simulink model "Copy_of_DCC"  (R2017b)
settings: Solver=FixedStepDiscrete  StartTime=0.0  StopTime=10.0  FixedStep=0.01  RelTol=1e-3  EnableMultiTasking=on
undefined symbols (not defined in the file): ASWTYPE_FALSE, ASWTYPE_TRUE, CbDCC_BMTMsgCmd_flg, CbDCC_BMVMsgCmd_flg, CbDCC_BSPMsgCmd_flg, CcDCC_BSTSendTi_ms, CcDCC_BulkSOC_pct, CcDCC_CCSTout_ms, CcDCC_CellTempFilterAvg_numb, CcDCC_ChrgCrnt0HysVolt_mV, CcDCC_ChrgFinOverTi_ms, CcDCC_ChrgMaxPackVoltLimt_V, CcDCC_ChrgSt2StepChrgTime_ms, CcDCC_ChrgStCutoffTime_ms, CcDCC_ChrgStFullChrgCrnt_A, CcDCC_CMLTout_ms, CcDCC_CommToutOverTi_ms, CcDCC_CRMAATout_ms, CcDCC_CRMCHMTout_ms, CcDCC_CRMTout_ms, CcDCC_CROAATout_ms, CcDCC_CROTout_ms, CcDCC_CSDTout_ms, CcDCC_CSTTout_ms, CcDCC_DC12VUnonnectTi_ms, CcDCC_DCChrgDispSOCPrmt_pct, CcDCC_DCChrgMismatch_ms, CcDCC_DCChrgPermitCfg_ms, CcDCC_DCChrgPrmtFltLvl_numb, CcDCC_DCChrgPrmtStop_ms, CcDCC_DCChrgStepCurr_A, CcDCC_DCChrgStop_ms, CcDCC_DCCrntUnctrolTi_ms, CcDCC_DCFullChrgHysVolt_mV, CcDCC_DCFullStepChrgTi1_ms, CcDCC_DCFullStepChrgTi2_ms, CcDCC_DCMaxChrgCurr_A, CcDCC_DCStepChrgWaitTime_ms, CcDCC_DCStop2DefaultTi_ms, CcDCC_DefaultWaitTi_ms, CcDCC_DiffDCChrgCrnt_A, CcDCC_DiffDCChrgCrntTi_ms, CcDCC_HeatChrgCrnt0Time_ms, CcDCC_HeatChrgCrnt1Time_ms, CcDCC_IsoDisableDelay_ms, CcDCC_MaxPackVoltLimt_V, CcDCC_SafeCur_A, CcDCC_StartChrgHysVolt_mV, CcDCC_StartDCChrgCellTemp_C, CcDCC_StepChrgCutoffTi_ms, CcDCC_StepChrgFullChrgCrnt_A, CcDCC_ToutDelay_ms, CcDCC_VehSpdFld_kmh, DCC_CONST0_NUMB, DCC_CONST1000_NUMB, DCC_CONST170_NUMB, DCC_RUNTIME_MS, Enum_BTMHeatReq, Enum_CTCCtrCtlConnMode, Enum_CTCCtrCtlState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
libraries: AIWAYS_Powertrain_BMS_lib x82
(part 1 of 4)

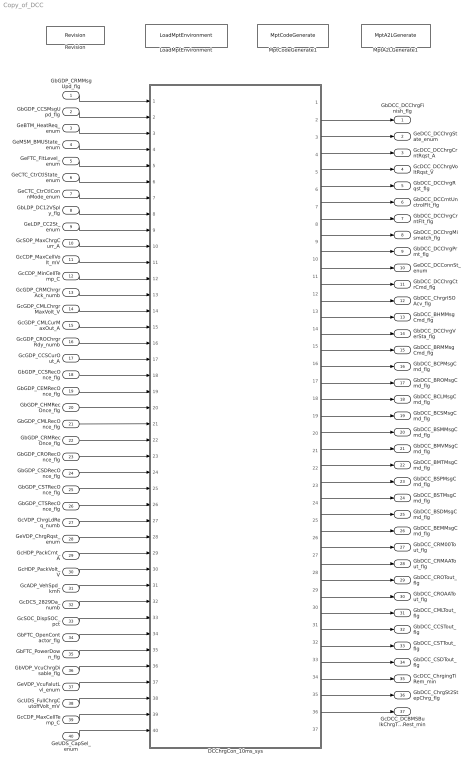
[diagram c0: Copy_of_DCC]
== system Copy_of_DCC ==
  GbGDP_CRMMsgUpd_flg : Inport
  GbGDP_CCSMsgUpd_flg : Inport  Port=2
  GeBTM_HeatReq_enum : Inport  Port=3
  GeMSM_BMUState_enum : Inport  Port=4
  GeFTC_FltLevel_enum : Inport  Port=5
  GeCTC_CtrCtlState_enum : Inport  Port=6
  GeCTC_CtrCtlConnMode_enum : Inport  Port=7
  GbLDP_DC12VSply_flg : Inport  Port=8
  GeLDP_CC2St_enum : Inport  Port=9
  GcSOP_MaxChrgCurr_A : Inport  Port=10
  GcCDP_MaxCellVolt_mV : Inport  Port=11
  GcCDP_MinCellTemp_C : Inport  Port=12
  GcGDP_CRMChrgrAck_numb : Inport  Port=13
  GcGDP_CMLChrgrMaxVolt_V : Inport  Port=14
  GcGDP_CMLCurMaxOut_A : Inport  Port=15
  GcGDP_CROChrgrRdy_numb : Inport  Port=16
  GcGDP_CCSCurOut_A : Inport  Port=17
  GbGDP_CCSRecOnce_flg : Inport  Port=18
  GbGDP_CEMRecOnce_flg : Inport  Port=19
  GbGDP_CHMRecOnce_flg : Inport  Port=20
  GbGDP_CMLRecOnce_flg : Inport  Port=21
  GbGDP_CRMRecOnce_flg : Inport  Port=22
  GbGDP_CRORecOnce_flg : Inport  Port=23
  GbGDP_CSDRecOnce_flg : Inport  Port=24
  GbGDP_CSTRecOnce_flg : Inport  Port=25
  GbGDP_CTSRecOnce_flg : Inport  Port=26
  GcVDP_ChrgLdReq_numb : Inport  Port=27
  GeVDP_ChrgRqst_enum : Inport  Port=28
  GcHDP_PackCrnt_A : Inport  Port=29
  GcHDP_PackVolt_V : Inport  Port=30
  GcADP_VehSpd_kmh : Inport  Port=31
  GcDCS_2829Da_numb : Inport  Port=32
  GcSOC_DispSOC_pct : Inport  Port=33
  GbFTC_OpenContactor_flg : Inport  Port=34
  GbFTC_PowerDown_flg : Inport  Port=35
  GbVDP_VcuChrgDisable_flg : Inport  Port=36
  GeVDP_VcuFalutLvl_enum : Inport  Port=37
  GcUDS_FullChrgCutoffVolt_mV : Inport  Port=38
  GcCDP_MaxCellTemp_C : Inport  Port=39
  GeUDS_CapSel_enum : Inport  Port=40
  DCChrgCon_10ms_sys : Subsystem
  LoadMptEnvironment : AIWAYS_Powertrain_BMS_lib/Config/LoadMptEnvironment  ProjectName=Comm  SuppierID=NewPlatformUAES
  MptA2LGenerate1 : AIWAYS_Powertrain_BMS_lib/Config/MptA2LGenerate  SystemSampleTime=-1
  MptCodeGenerate1 : AIWAYS_Powertrain_BMS_lib/Config/MptCodeGenerate  SystemSampleTime=-1
  Revision : AIWAYS_Powertrain_BMS_lib/Config/Revision  curVersion='M111C107'  newVersion='M112C107'
  GbDCC_DCChrgFinish_flg : Outport
  GeDCC_DCChrgState_enum : Outport  Port=2
  GcDCC_DCChrgCrntRqst_A : Outport  Port=3
  GcDCC_DCChrgVoltRqst_V : Outport  Port=4
  GbDCC_DCChrgRqst_flg : Outport  Port=5
  GbDCC_DCCrntUnctrolFlt_flg : Outport  Port=6
  GbDCC_DCChrgCrntFlt_flg : Outport  Port=7
  GbDCC_DCChrgMismatch_flg : Outport  Port=8
  GbDCC_DCChrgPrmt_flg : Outport  Port=9
  GeDCC_DCConnSt_enum : Outport  Port=10
  GbDCC_DCChrgCtrCmd_flg : Outport  Port=11
  GbDCC_ChrgrISOAcv_flg : Outport  Port=12
  GbDCC_BHMMsgCmd_flg : Outport  Port=13
  GbDCC_DCChrgVerSta_flg : Outport  Port=14
  GbDCC_BRMMsgCmd_flg : Outport  Port=15
  GbDCC_BCPMsgCmd_flg : Outport  Port=16
  GbDCC_BROMsgCmd_flg : Outport  Port=17
  GbDCC_BCLMsgCmd_flg : Outport  Port=18
  GbDCC_BCSMsgCmd_flg : Outport  Port=19
  GbDCC_BSMMsgCmd_flg : Outport  Port=20
  GbDCC_BMVMsgCmd_flg : Outport  Port=21
  GbDCC_BMTMsgCmd_flg : Outport  Port=22
  GbDCC_BSPMsgCmd_flg : Outport  Port=23
  GbDCC_BSTMsgCmd_flg : Outport  Port=24
  GbDCC_BSDMsgCmd_flg : Outport  Port=25
  GbDCC_BEMMsgCmd_flg : Outport  Port=26
  GbDCC_CRM00Tout_flg : Outport  Port=27
  GbDCC_CRMAATout_flg : Outport  Port=28
  GbDCC_CROTout_flg : Outport  Port=29
  GbDCC_CROAATout_flg : Outport  Port=30
  GbDCC_CMLTout_flg : Outport  Port=31
  GbDCC_CCSTout_flg : Outport  Port=32
  GbDCC_CSTTout_flg : Outport  Port=33
  GbDCC_CSDTout_flg : Outport  Port=34
  GcDCC_ChrgingTiRem_min : Outport  Port=35
  GbDCC_ChrgSt2StepChrg_flg : Outport  Port=36
  GcDCC_DCBMSBulkChrgTimeRest_min : Outport  Port=37
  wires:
  DCChrgCon_10ms_sys/1(GbDCC_DCChrgFinish_flg) -> GbDCC_DCChrgFinish_flg/1
  DCChrgCon_10ms_sys/3(GcDCC_DCChrgCrntRqst_A) -> GcDCC_DCChrgCrntRqst_A/1
  DCChrgCon_10ms_sys/2(GeDCC_DCChrgState_enum) -> GeDCC_DCChrgState_enum/1
  DCChrgCon_10ms_sys/7(GbDCC_DCChrgCrntFlt_flg) -> GbDCC_DCChrgCrntFlt_flg/1
  DCChrgCon_10ms_sys/4(GcDCC_DCChrgVoltRqst_V) -> GcDCC_DCChrgVoltRqst_V/1
  DCChrgCon_10ms_sys/10(GeDCC_DCConnSt_enum) -> GeDCC_DCConnSt_enum/1
  DCChrgCon_10ms_sys/12(GbDCC_ChrgrISOAcv_flg) -> GbDCC_ChrgrISOAcv_flg/1
  DCChrgCon_10ms_sys/15(GbDCC_BRMMsgCmd_flg) -> GbDCC_BRMMsgCmd_flg/1
  DCChrgCon_10ms_sys/16(GbDCC_BCPMsgCmd_flg) -> GbDCC_BCPMsgCmd_flg/1
  GeLDP_CC2St_enum/1 -> DCChrgCon_10ms_sys/9(GeLDP_CC2St_enum)
  DCChrgCon_10ms_sys/11(GbDCC_DCChrgCtrCmd_flg) -> GbDCC_DCChrgCtrCmd_flg/1
  GcSOP_MaxChrgCurr_A/1 -> DCChrgCon_10ms_sys/10(GcSOP_MaxChrgCurr_A)
  GcCDP_MinCellTemp_C/1 -> DCChrgCon_10ms_sys/12(GcCDP_MinCellTemp_C)
  GcGDP_CMLChrgrMaxVolt_V/1 -> DCChrgCon_10ms_sys/14(GcGDP_CMLChrgrMaxVolt_V)
  GeBTM_HeatReq_enum/1 -> DCChrgCon_10ms_sys/3(GeBTM_HeatReq_enum)
  DCChrgCon_10ms_sys/5(GbDCC_DCChrgRqst_flg) -> GbDCC_DCChrgRqst_flg/1
  DCChrgCon_10ms_sys/25(GbDCC_BSDMsgCmd_flg) -> GbDCC_BSDMsgCmd_flg/1
  GeUDS_CapSel_enum/1 -> DCChrgCon_10ms_sys/40(GeUDS_CapSel_enum)
  GcGDP_CROChrgrRdy_numb/1 -> DCChrgCon_10ms_sys/16(GcGDP_CROChrgrRdy_numb)
  GbGDP_CRMMsgUpd_flg/1 -> DCChrgCon_10ms_sys/1(GbGDP_CRMMsgUpd_flg)
  DCChrgCon_10ms_sys/22(GbDCC_BMTMsgCmd_flg) -> GbDCC_BMTMsgCmd_flg/1
  GcGDP_CCSCurOut_A/1 -> DCChrgCon_10ms_sys/17(GcGDP_CCSCurOut_A)
  DCChrgCon_10ms_sys/30(GbDCC_CROAATout_flg) -> GbDCC_CROAATout_flg/1
  GbGDP_CMLRecOnce_flg/1 -> DCChrgCon_10ms_sys/21(GbGDP_CMLRecOnce_flg)
  DCChrgCon_10ms_sys/14(GbDCC_DCChrgVerSta_flg) -> GbDCC_DCChrgVerSta_flg/1
  GbGDP_CRORecOnce_flg/1 -> DCChrgCon_10ms_sys/23(GbGDP_CRORecOnce_flg)
  DCChrgCon_10ms_sys/32(GbDCC_CCSTout_flg) -> GbDCC_CCSTout_flg/1
  DCChrgCon_10ms_sys/17(GbDCC_BROMsgCmd_flg) -> GbDCC_BROMsgCmd_flg/1
  GeFTC_FltLevel_enum/1 -> DCChrgCon_10ms_sys/5(GeFTC_FltLevel_enum)
  DCChrgCon_10ms_sys/27(GbDCC_CRM00Tout_flg) -> GbDCC_CRM00Tout_flg/1
  DCChrgCon_10ms_sys/13(GbDCC_BHMMsgCmd_flg) -> GbDCC_BHMMsgCmd_flg/1
  DCChrgCon_10ms_sys/28(GbDCC_CRMAATout_flg) -> GbDCC_CRMAATout_flg/1
  GcCDP_MaxCellVolt_mV/1 -> DCChrgCon_10ms_sys/11(GcCDP_MaxCellVolt_mV)
  GbLDP_DC12VSply_flg/1 -> DCChrgCon_10ms_sys/8(GbLDP_DC12VSply_flg)
  DCChrgCon_10ms_sys/20(GbDCC_BSMMsgCmd_flg) -> GbDCC_BSMMsgCmd_flg/1
  DCChrgCon_10ms_sys/24(GbDCC_BSTMsgCmd_flg) -> GbDCC_BSTMsgCmd_flg/1
  GeVDP_VcuFalutLvl_enum/1 -> DCChrgCon_10ms_sys/37(GeVDP_VcuFalutLvl_enum)
  GcVDP_ChrgLdReq_numb/1 -> DCChrgCon_10ms_sys/27(GcVDP_ChrgLdReq_numb)
  GcHDP_PackCrnt_A/1 -> DCChrgCon_10ms_sys/29(GcHDP_PackCrnt_A)
  GcCDP_MaxCellTemp_C/1 -> DCChrgCon_10ms_sys/39(GcCDP_MaxCellTemp_C)
  GbGDP_CCSRecOnce_flg/1 -> DCChrgCon_10ms_sys/18(GbGDP_CCSRecOnce_flg)
  GcDCS_2829Da_numb/1 -> DCChrgCon_10ms_sys/32(GcDCS_2829Da_numb)
  GcADP_VehSpd_kmh/1 -> DCChrgCon_10ms_sys/31(GcADP_VehSpd_kmh)
  DCChrgCon_10ms_sys/37(GcDCC_DCBMSBulkChrgTimeRest_min) -> GcDCC_DCBMSBulkChrgTimeRest_min/1
  DCChrgCon_10ms_sys/23(GbDCC_BSPMsgCmd_flg) -> GbDCC_BSPMsgCmd_flg/1
  GbGDP_CSTRecOnce_flg/1 -> DCChrgCon_10ms_sys/25(GbGDP_CSTRecOnce_flg)
  DCChrgCon_10ms_sys/21(GbDCC_BMVMsgCmd_flg) -> GbDCC_BMVMsgCmd_flg/1
  GcSOC_DispSOC_pct/1 -> DCChrgCon_10ms_sys/33(GcSOC_DispSOC_pct)
  DCChrgCon_10ms_sys/9(GbDCC_DCChrgPrmt_flg) -> GbDCC_DCChrgPrmt_flg/1
  GcUDS_FullChrgCutoffVolt_mV/1 -> DCChrgCon_10ms_sys/38(GcUDS_FullChrgCutoffVolt_mV)
  DCChrgCon_10ms_sys/35(GcDCC_ChrgingTiRem_min) -> GcDCC_ChrgingTiRem_min/1
  DCChrgCon_10ms_sys/36(GbDCC_ChrgSt2StepChrg_flg) -> GbDCC_ChrgSt2StepChrg_flg/1
  GeVDP_ChrgRqst_enum/1 -> DCChrgCon_10ms_sys/28(GeVDP_ChrgRqst_enum)
  GbGDP_CRMRecOnce_flg/1 -> DCChrgCon_10ms_sys/22(GbGDP_CRMRecOnce_flg)
  GcHDP_PackVolt_V/1 -> DCChrgCon_10ms_sys/30(GcHDP_PackVolt_V)
  DCChrgCon_10ms_sys/31(GbDCC_CMLTout_flg) -> GbDCC_CMLTout_flg/1
  GbGDP_CEMRecOnce_flg/1 -> DCChrgCon_10ms_sys/19(GbGDP_CEMRecOnce_flg)
  GeCTC_CtrCtlState_enum/1 -> DCChrgCon_10ms_sys/6(GeCTC_CtrCtlState_enum)
  GbGDP_CCSMsgUpd_flg/1 -> DCChrgCon_10ms_sys/2(GbGDP_CCSMsgUpd_flg)
  GbFTC_PowerDown_flg/1 -> DCChrgCon_10ms_sys/35(GbFTC_PowerDown_flg)
  DCChrgCon_10ms_sys/26(GbDCC_BEMMsgCmd_flg) -> GbDCC_BEMMsgCmd_flg/1
  GbGDP_CSDRecOnce_flg/1 -> DCChrgCon_10ms_sys/24(GbGDP_CSDRecOnce_flg)
  GbGDP_CTSRecOnce_flg/1 -> DCChrgCon_10ms_sys/26(GbGDP_CTSRecOnce_flg)
  GcGDP_CMLCurMaxOut_A/1 -> DCChrgCon_10ms_sys/15(GcGDP_CMLCurMaxOut_A)
  GbGDP_CHMRecOnce_flg/1 -> DCChrgCon_10ms_sys/20(GbGDP_CHMRecOnce_flg)
  DCChrgCon_10ms_sys/6(GbDCC_DCCrntUnctrolFlt_flg) -> GbDCC_DCCrntUnctrolFlt_flg/1
  DCChrgCon_10ms_sys/29(GbDCC_CROTout_flg) -> GbDCC_CROTout_flg/1
  DCChrgCon_10ms_sys/34(GbDCC_CSDTout_flg) -> GbDCC_CSDTout_flg/1
  GbVDP_VcuChrgDisable_flg/1 -> DCChrgCon_10ms_sys/36(GbVDP_VcuChrgDisable_flg)
  DCChrgCon_10ms_sys/19(GbDCC_BCSMsgCmd_flg) -> GbDCC_BCSMsgCmd_flg/1
  GeCTC_CtrCtlConnMode_enum/1 -> DCChrgCon_10ms_sys/7(GeCTC_CtrCtlConnMode_enum)
  DCChrgCon_10ms_sys/18(GbDCC_BCLMsgCmd_flg) -> GbDCC_BCLMsgCmd_flg/1
  GeMSM_BMUState_enum/1 -> DCChrgCon_10ms_sys/4(GeMSM_BMUState_enum)
  GbFTC_OpenContactor_flg/1 -> DCChrgCon_10ms_sys/34(GbFTC_OpenContactor_flg)
  GcGDP_CRMChrgrAck_numb/1 -> DCChrgCon_10ms_sys/13(GcGDP_CRMChrgrAck_numb)
  DCChrgCon_10ms_sys/33(GbDCC_CSTTout_flg) -> GbDCC_CSTTout_flg/1
  DCChrgCon_10ms_sys/8(GbDCC_DCChrgMismatch_flg) -> GbDCC_DCChrgMismatch_flg/1

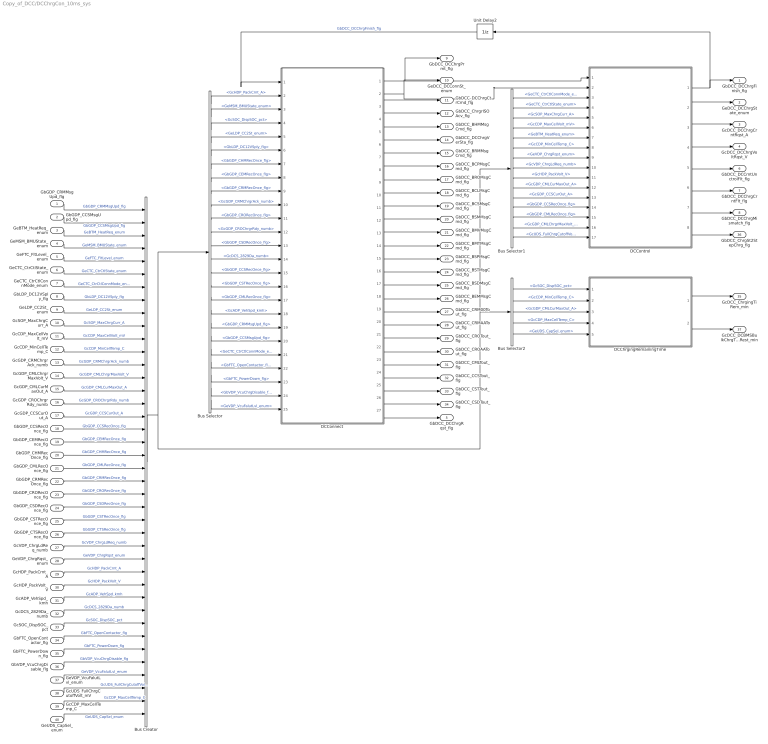
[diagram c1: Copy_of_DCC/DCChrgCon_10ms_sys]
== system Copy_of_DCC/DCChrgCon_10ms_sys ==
  GbGDP_CRMMsgUpd_flg : Inport
  GbGDP_CCSMsgUpd_flg : Inport  Port=2
  GeBTM_HeatReq_enum : Inport  Port=3
  GeMSM_BMUState_enum : Inport  Port=4
  GeFTC_FltLevel_enum : Inport  Port=5
  GeCTC_CtrCtlState_enum : Inport  Port=6
  GeCTC_CtrCtlConnMode_enum : Inport  Port=7
  GbLDP_DC12VSply_flg : Inport  Port=8
  GeLDP_CC2St_enum : Inport  Port=9
  GcSOP_MaxChrgCurr_A : Inport  Port=10
  GcCDP_MaxCellVolt_mV : Inport  Port=11
  GcCDP_MinCellTemp_C : Inport  Port=12
  GcGDP_CRMChrgrAck_numb : Inport  Port=13
  GcGDP_CMLChrgrMaxVolt_V : Inport  Port=14
  GcGDP_CMLCurMaxOut_A : Inport  Port=15
  GcGDP_CROChrgrRdy_numb : Inport  Port=16
  GcGDP_CCSCurOut_A : Inport  Port=17
  GbGDP_CCSRecOnce_flg : Inport  Port=18
  GbGDP_CEMRecOnce_flg : Inport  Port=19
  GbGDP_CHMRecOnce_flg : Inport  Port=20
  GbGDP_CMLRecOnce_flg : Inport  Port=21
  GbGDP_CRMRecOnce_flg : Inport  Port=22
  GbGDP_CRORecOnce_flg : Inport  Port=23
  GbGDP_CSDRecOnce_flg : Inport  Port=24
  GbGDP_CSTRecOnce_flg : Inport  Port=25
  GbGDP_CTSRecOnce_flg : Inport  Port=26
  GcVDP_ChrgLdReq_numb : Inport  Port=27
  GeVDP_ChrgRqst_enum : Inport  Port=28
  GcHDP_PackCrnt_A : Inport  Port=29
  GcHDP_PackVolt_V : Inport  Port=30
  GcADP_VehSpd_kmh : Inport  Port=31
  GcDCS_2829Da_numb : Inport  Port=32
  GcSOC_DispSOC_pct : Inport  Port=33
  GbFTC_OpenContactor_flg : Inport  Port=34
  GbFTC_PowerDown_flg : Inport  Port=35
  GbVDP_VcuChrgDisable_flg : Inport  Port=36
  GeVDP_VcuFalutLvl_enum : Inport  Port=37
  GcUDS_FullChrgCutoffVolt_mV : Inport  Port=38
  GcCDP_MaxCellTemp_C : Inport  Port=39
  GeUDS_CapSel_enum : Inport  Port=40
  Bus Creator : BusCreator  Inputs=40
  Bus Selector : BusSelector  OutputSignals=GcHDP_PackCrnt_A,GeMSM_BMUState_enum,GcSOC_DispSOC_pct,GeLDP_CC2St_enum,GbLDP_DC12VSply_flg,GbGDP_CHMRecOnce_flg,GbGDP_CEMRecOnce_flg,GbGDP_CRMRecOnce_flg,GcGDP_CRMChrgrAck_numb,GbGDP_CRORecOnce_flg,GcGDP_CROChrgrRdy_numb,GbGDP_CSDRecOnce_flg,GcDCS_2829Da_numb,GbGDP_CCSRecOnce_flg,GbGDP_CSTRecOnce_flg,GbGDP_CMLRecOnce_flg,GcADP_VehSpd_kmh,GbGDP_CRMMsgUpd_flg,GbGDP_CCSMsgUpd_flg,GeCTC_CtrCtlConnMod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
  Bus Selector1 : BusSelector  OutputSignals=GeCTC_CtrCtlConnMode_enum,GeCTC_CtrCtlState_enum,GcSOP_MaxChrgCurr_A,GcCDP_MaxCellVolt_mV,GeBTM_HeatReq_enum,GcCDP_MinCellTemp_C,GeVDP_ChrgRqst_enum,GcVDP_ChrgLdReq_numb,GcHDP_PackVolt_V,GcGDP_CMLCurMaxOut_A,GcGDP_CCSCurOut_A,GbGDP_CCSRecOnce_flg,GbGDP_CMLRecOnce_flg,GcGDP_CMLChrgrMaxVolt_V,GcUDS_FullChrgCutoffVolt_mV
  Bus Selector2 : BusSelector  OutputSignals=GcSOC_DispSOC_pct,GcCDP_MinCellTemp_C,GcGDP_CMLCurMaxOut_A,GcCDP_MaxCellTemp_C,GeUDS_CapSel_enum
  DCChrgingRemainingTime : Subsystem
  DCConnect : Subsystem
  DCControl : Subsystem
  Unit Delay2 : UnitDelay  SampleTime=-1  StateName=StateName
  GbDCC_DCChrgFinish_flg : Outport
  GeDCC_DCChrgState_enum : Outport  Port=2
  GcDCC_DCChrgCrntRqst_A : Outport  Port=3
  GcDCC_DCChrgVoltRqst_V : Outport  Port=4
  GbDCC_DCChrgRqst_flg : Outport  Port=5
  GbDCC_DCCrntUnctrolFlt_flg : Outport  Port=6
  GbDCC_DCChrgCrntFlt_flg : Outport  Port=7
  GbDCC_DCChrgMismatch_flg : Outport  Port=8
  GbDCC_DCChrgPrmt_flg : Outport  Port=9
  GeDCC_DCConnSt_enum : Outport  Port=10
  GbDCC_DCChrgCtrCmd_flg : Outport  Port=11
  GbDCC_ChrgrISOAcv_flg : Outport  Port=12
  GbDCC_BHMMsgCmd_flg : Outport  Port=13
  GbDCC_DCChrgVerSta_flg : Outport  Port=14
  GbDCC_BRMMsgCmd_flg : Outport  Port=15
  GbDCC_BCPMsgCmd_flg : Outport  Port=16
  GbDCC_BROMsgCmd_flg : Outport  Port=17
  GbDCC_BCLMsgCmd_flg : Outport  Port=18
  GbDCC_BCSMsgCmd_flg : Outport  Port=19
  GbDCC_BSMMsgCmd_flg : Outport  Port=20
  GbDCC_BMVMsgCmd_flg : Outport  Port=21
  GbDCC_BMTMsgCmd_flg : Outport  Port=22
  GbDCC_BSPMsgCmd_flg : Outport  Port=23
  GbDCC_BSTMsgCmd_flg : Outport  Port=24
  GbDCC_BSDMsgCmd_flg : Outport  Port=25
  GbDCC_BEMMsgCmd_flg : Outport  Port=26
  GbDCC_CRM00Tout_flg : Outport  Port=27
  GbDCC_CRMAATout_flg : Outport  Port=28
  GbDCC_CROTout_flg : Outport  Port=29
  GbDCC_CROAATout_flg : Outport  Port=30
  GbDCC_CMLTout_flg : Outport  Port=31
  GbDCC_CCSTout_flg : Outport  Port=32
  GbDCC_CSTTout_flg : Outport  Port=33
  GbDCC_CSDTout_flg : Outport  Port=34
  GcDCC_ChrgingTiRem_min : Outport  Port=35
  GbDCC_ChrgSt2StepChrg_flg : Outport  Port=36
  GcDCC_DCBMSBulkChrgTimeRest_min : Outport  Port=37
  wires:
  GbGDP_CRMMsgUpd_flg/1 -> Bus Creator/1  "GbGDP_CRMMsgUpd_flg"
  GbGDP_CCSMsgUpd_flg/1 -> Bus Creator/2  "GbGDP_CCSMsgUpd_flg"
  GeBTM_HeatReq_enum/1 -> Bus Creator/3  "GeBTM_HeatReq_enum"
  GeMSM_BMUState_enum/1 -> Bus Creator/4  "GeMSM_BMUState_enum"
  GeFTC_FltLevel_enum/1 -> Bus Creator/5  "GeFTC_FltLevel_enum"
  GeCTC_CtrCtlState_enum/1 -> Bus Creator/6  "GeCTC_CtrCtlState_enum"
  GeCTC_CtrCtlConnMode_enum/1 -> Bus Creator/7  "GeCTC_CtrCtlConnMode_enum"
  GbLDP_DC12VSply_flg/1 -> Bus Creator/8  "GbLDP_DC12VSply_flg"
  GeLDP_CC2St_enum/1 -> Bus Creator/9  "GeLDP_CC2St_enum"
  GcSOP_MaxChrgCurr_A/1 -> Bus Creator/10  "GcSOP_MaxChrgCurr_A"
  GcCDP_MaxCellVolt_mV/1 -> Bus Creator/11  "GcCDP_MaxCellVolt_mV"
  GcCDP_MinCellTemp_C/1 -> Bus Creator/12  "GcCDP_MinCellTemp_C"
  GcGDP_CRMChrgrAck_numb/1 -> Bus Creator/13  "GcGDP_CRMChrgrAck_numb"
  GcGDP_CMLChrgrMaxVolt_V/1 -> Bus Creator/14  "GcGDP_CMLChrgrMaxVolt_V"
  GcGDP_CMLCurMaxOut_A/1 -> Bus Creator/15  "GcGDP_CMLCurMaxOut_A"
  GcGDP_CROChrgrRdy_numb/1 -> Bus Creator/16  "GcGDP_CROChrgrRdy_numb"
  GcGDP_CCSCurOut_A/1 -> Bus Creator/17  "GcGDP_CCSCurOut_A"
  GbGDP_CCSRecOnce_flg/1 -> Bus Creator/18  "GbGDP_CCSRecOnce_flg"
  GbGDP_CEMRecOnce_flg/1 -> Bus Creator/19  "GbGDP_CEMRecOnce_flg"
  GbGDP_CHMRecOnce_flg/1 -> Bus Creator/20  "GbGDP_CHMRecOnce_flg"
  GbGDP_CMLRecOnce_flg/1 -> Bus Creator/21  "GbGDP_CMLRecOnce_flg"
  GbGDP_CRMRecOnce_flg/1 -> Bus Creator/22  "GbGDP_CRMRecOnce_flg"
  GbGDP_CRORecOnce_flg/1 -> Bus Creator/23  "GbGDP_CRORecOnce_flg"
  GbGDP_CSDRecOnce_flg/1 -> Bus Creator/24  "GbGDP_CSDRecOnce_flg"
  GbGDP_CSTRecOnce_flg/1 -> Bus Creator/25  "GbGDP_CSTRecOnce_flg"
  GbGDP_CTSRecOnce_flg/1 -> Bus Creator/26  "GbGDP_CTSRecOnce_flg"
  GcVDP_ChrgLdReq_numb/1 -> Bus Creator/27  "GcVDP_ChrgLdReq_numb"
  GeVDP_ChrgRqst_enum/1 -> Bus Creator/28  "GeVDP_ChrgRqst_enum"
  GcHDP_PackCrnt_A/1 -> Bus Creator/29  "GcHDP_PackCrnt_A"
  GcHDP_PackVolt_V/1 -> Bus Creator/30  "GcHDP_PackVolt_V"
  GcADP_VehSpd_kmh/1 -> Bus Creator/31  "GcADP_VehSpd_kmh"
  GcDCS_2829Da_numb/1 -> Bus Creator/32  "GcDCS_2829Da_numb"
  Bus Creator/1 -> Bus Selector/1, Bus Selector1/1, Bus Selector2/1
  GcSOC_DispSOC_pct/1 -> Bus Creator/33  "GcSOC_DispSOC_pct"
  DCControl/2(GeDCC_DCChrgState_enum) -> GeDCC_DCChrgState_enum/1
  DCControl/3(GcDCC_DCChrgCrntRqst_A) -> GcDCC_DCChrgCrntRqst_A/1
  DCControl/4(GcDCC_DCChrgVoltRqst_V) -> GcDCC_DCChrgVoltRqst_V/1
  DCControl/5(GbDCC_DCCrntUnctrolFlt_flg) -> GbDCC_DCCrntUnctrolFlt_flg/1
  DCControl/6(GbDCC_DCChrgCrntFlt_flg) -> GbDCC_DCChrgCrntFlt_flg/1
  DCControl/7(GbDCC_DCChrgMismatch_flg) -> GbDCC_DCChrgMismatch_flg/1
  DCControl/1(GbDCC_DCChrgFinish_flg) -> Unit Delay2/1, GbDCC_DCChrgFinish_flg/1
  Bus Selector/1 -> DCConnect/2(GcHDP_PackCrnt_A)  "<GcHDP_PackCrnt_A>"
  Bus Selector/2 -> DCConnect/3(GeMSM_BMUState_enum)  "<GeMSM_BMUState_enum>"
  Bus Selector/3 -> DCConnect/4(GcSOC_DispSOC_pct)  "<GcSOC_DispSOC_pct>"
  Bus Selector/6 -> DCConnect/7(GbGDP_CHMRecOnce_flg)  "<GbGDP_CHMRecOnce_flg>"
  Bus Selector/7 -> DCConnect/8(GbGDP_CEMRecOnce_flg)  "<GbGDP_CEMRecOnce_flg>"
  Bus Selector/8 -> DCConnect/9(GbGDP_CRMRecOnce_flg)  "<GbGDP_CRMRecOnce_flg>"
  Bus Selector/9 -> DCConnect/10(GcGDP_CRMChrgrAck_numb)  "<GcGDP_CRMChrgrAck_numb>"
  Bus Selector/10 -> DCConnect/11(GbGDP_CRORecOnce_flg)  "<GbGDP_CRORecOnce_flg>"
  Bus Selector/11 -> DCConnect/12(GcGDP_CROChrgrRdy_numb)  "<GcGDP_CROChrgrRdy_numb>"
  Bus Selector/12 -> DCConnect/13(GbGDP_CSDRecOnce_flg)  "<GbGDP_CSDRecOnce_flg>"
  Bus Selector/13 -> DCConnect/14(GcDCS_2829Da_numb)  "<GcDCS_2829Da_numb>"
  Bus Selector/14 -> DCConnect/15(GbGDP_CCSRecOnce_flg)  "<GbGDP_CCSRecOnce_flg>"
  Bus Selector/15 -> DCConnect/16(GbGDP_CSTRecOnce_flg)  "<GbGDP_CSTRecOnce_flg>"
  Bus Selector/16 -> DCConnect/17(GbGDP_CMLRecOnce_flg)  "<GbGDP_CMLRecOnce_flg>"
  Bus Selector/17 -> DCConnect/18(GcADP_VehSpd_kmh)  "<GcADP_VehSpd_kmh>"
  Bus Selector/18 -> DCConnect/19(GbGDP_CRMMsgUpd_flg)  "<GbGDP_CRMMsgUpd_flg>"
  Bus Selector/19 -> DCConnect/20(GbGDP_CCSMsgUpd_flg)  "<GbGDP_CCSMsgUpd_flg>"
  DCConnect/1(GbDCC_DCChrgPrmt_flg) -> GbDCC_DCChrgPrmt_flg/1, DCControl/1(GbDCC_DCChrgPrmt_flg)
  DCConnect/2(GeDCC_DCConnSt_enum) -> GeDCC_DCConnSt_enum/1, DCControl/2(GeDCC_DCConnSt_enum)
  Bus Selector1/1 -> DCControl/3(GeCTC_CtrCtlConnMode_enum)  "<GeCTC_CtrCtlConnMode_enum>"
  Bus Selector1/2 -> DCControl/4(GeCTC_CtrCtlState_enum)  "<GeCTC_CtrCtlState_enum>"
  Bus Selector1/3 -> DCControl/5(GcSOP_MaxChrgCurr_A)  "<GcSOP_MaxChrgCurr_A>"
  Bus Selector1/4 -> DCControl/6(GcCDP_MaxCellVolt_mV)  "<GcCDP_MaxCellVolt_mV>"
  Bus Selector1/5 -> DCControl/7(GeBTM_HeatReq_enum)  "<GeBTM_HeatReq_enum>"
  Bus Selector1/6 -> DCControl/8(GcCDP_MinCellTemp_C)  "<GcCDP_MinCellTemp_C>"
  Bus Selector1/7 -> DCControl/9(GeVDP_ChrgRqst_enum)  "<GeVDP_ChrgRqst_enum>"
  Bus Selector1/8 -> DCControl/10(GcVDP_ChrgLdReq_numb)  "<GcVDP_ChrgLdReq_numb>"
  Bus Selector1/9 -> DCControl/11(GcHDP_PackVolt_V)  "<GcHDP_PackVolt_V>"
  Bus Selector1/10 -> DCControl/12(GcGDP_CMLCurMaxOut_A)  "<GcGDP_CMLCurMaxOut_A>"
  Bus Selector1/11 -> DCControl/13(GcGDP_CCSCurOut_A)  "<GcGDP_CCSCurOut_A>"
  Bus Selector1/12 -> DCControl/14(GbGDP_CCSRecOnce_flg)  "<GbGDP_CCSRecOnce_flg>"
  Bus Selector1/13 -> DCControl/15(GbGDP_CMLRecOnce_flg)  "<GbGDP_CMLRecOnce_flg>"
  Bus Selector1/14 -> DCControl/16(GcGDP_CMLChrgrMaxVolt_V)  "<GcGDP_CMLChrgrMaxVolt_V>"
  DCConnect/3(GbDCC_DCChrgCtrCmd_flg) -> GbDCC_DCChrgCtrCmd_flg/1
  DCConnect/4(GbDCC_ChrgrISOAcv_flg) -> GbDCC_ChrgrISOAcv_flg/1
  DCConnect/5(GbDCC_BHMMsgCmd_flg) -> GbDCC_BHMMsgCmd_flg/1
  DCConnect/6(GbDCC_DCChrgVerSta_flg) -> GbDCC_DCChrgVerSta_flg/1
  DCConnect/7(GbDCC_BRMMsgCmd_flg) -> GbDCC_BRMMsgCmd_flg/1
  DCConnect/8(GbDCC_BCPMsgCmd_flg) -> GbDCC_BCPMsgCmd_flg/1
  DCConnect/9(GbDCC_BROMsgCmd_flg) -> GbDCC_BROMsgCmd_flg/1
  DCConnect/10(GbDCC_BCLMsgCmd_flg) -> GbDCC_BCLMsgCmd_flg/1
  DCConnect/11(GbDCC_BCSMsgCmd_flg) -> GbDCC_BCSMsgCmd_flg/1
  DCConnect/12(GbDCC_BSMMsgCmd_flg) -> GbDCC_BSMMsgCmd_flg/1
  DCConnect/13(GbDCC_BMVMsgCmd_flg) -> GbDCC_BMVMsgCmd_flg/1
  DCConnect/14(GbDCC_BMTMsgCmd_flg) -> GbDCC_BMTMsgCmd_flg/1
  DCConnect/15(GbDCC_BSPMsgCmd_flg) -> GbDCC_BSPMsgCmd_flg/1
  DCConnect/16(GbDCC_BSTMsgCmd_flg) -> GbDCC_BSTMsgCmd_flg/1
  DCConnect/17(GbDCC_BSDMsgCmd_flg) -> GbDCC_BSDMsgCmd_flg/1
  DCConnect/18(GbDCC_BEMMsgCmd_flg) -> GbDCC_BEMMsgCmd_flg/1
  DCConnect/19(GbDCC_CRM00Tout_flg) -> GbDCC_CRM00Tout_flg/1
  DCConnect/20(GbDCC_CRMAATout_flg) -> GbDCC_CRMAATout_flg/1
  DCConnect/21(GbDCC_CROTout_flg) -> GbDCC_CROTout_flg/1
  DCConnect/22(GbDCC_CROAATout_flg) -> GbDCC_CROAATout_flg/1
  DCConnect/23(GbDCC_CMLTout_flg) -> GbDCC_CMLTout_flg/1
  DCConnect/24(GbDCC_CCSTout_flg) -> GbDCC_CCSTout_flg/1
  DCConnect/25(GbDCC_CSTTout_flg) -> GbDCC_CSTTout_flg/1
  DCConnect/26(GbDCC_CSDTout_flg) -> GbDCC_CSDTout_flg/1
  Bus Selector/4 -> DCConnect/5(GeLDP_CC2St_enum)  "<GeLDP_CC2St_enum>"
  Bus Selector/5 -> DCConnect/6(GbLDP_DC12VSply_flg)  "<GbLDP_DC12VSply_flg>"
  Unit Delay2/1 -> DCConnect/1(GbDCC_DCChrgFinish_flg)  "GbDCC_DCChrgFinish_flg"
  DCChrgingRemainingTime/1(GcDCC_ChrgingTiRem_min) -> GcDCC_ChrgingTiRem_min/1
  Bus Selector/20 -> DCConnect/21(GeCTC_CtrCtlConnMode_enum)  "<GeCTC_CtrCtlConnMode_enum>"
  DCControl/8(GbDCC_ChrgSt2StepChrg_flg) -> GbDCC_ChrgSt2StepChrg_flg/1
  GbVDP_VcuChrgDisable_flg/1 -> Bus Creator/36  "GbVDP_VcuChrgDisable_flg"
  GbFTC_PowerDown_flg/1 -> Bus Creator/35  "GbFTC_PowerDown_flg"
  GbFTC_OpenContactor_flg/1 -> Bus Creator/34  "GbFTC_OpenContactor_flg"
  Bus Selector/21 -> DCConnect/22(GbFTC_OpenContactor_flg)  "<GbFTC_OpenContactor_flg>"
  Bus Selector/22 -> DCConnect/23(GbFTC_PowerDown_flg)  "<GbFTC_PowerDown_flg>"
  Bus Selector/23 -> DCConnect/24(GbVDP_VcuChrgDisable_flg)  "<GbVDP_VcuChrgDisable_flg>"
  GeVDP_VcuFalutLvl_enum/1 -> Bus Creator/37  "GeVDP_VcuFalutLvl_enum"
  Bus Selector/24 -> DCConnect/25(GeVDP_VcuFalutLvl_enum)  "<GeVDP_VcuFalutLvl_enum>"
  DCConnect/27(GbDCC_DCChrgRqst_flg) -> GbDCC_DCChrgRqst_flg/1
  GcUDS_FullChrgCutoffVolt_mV/1 -> Bus Creator/38  "GcUDS_FullChrgCutoffVolt_mV"
  Bus Selector1/15 -> DCControl/17(GcUDS_FullChrgCutoffVolt_mV)  "<GcUDS_FullChrgCutoffVolt_mV>"
  GcCDP_MaxCellTemp_C/1 -> Bus Creator/39  "GcCDP_MaxCellTemp_C"
  GeUDS_CapSel_enum/1 -> Bus Creator/40  "GeUDS_CapSel_enum"
  Bus Selector2/1 -> DCChrgingRemainingTime/1(GcSOC_DispSOC_pct)  "<GcSOC_DispSOC_pct>"
  Bus Selector2/2 -> DCChrgingRemainingTime/2(GcCDP_MinCellTemp_C)  "<GcCDP_MinCellTemp_C>"
  Bus Selector2/3 -> DCChrgingRemainingTime/3(GcGDP_CMLCurMaxOut_A)  "<GcGDP_CMLCurMaxOut_A>"
  Bus Selector2/4 -> DCChrgingRemainingTime/4(GcCDP_MaxCellTemp_C)  "<GcCDP_MaxCellTemp_C>"
  Bus Selector2/5 -> DCChrgingRemainingTime/5(GeUDS_CapSel_enum)  "<GeUDS_CapSel_enum>"
  DCChrgingRemainingTime/2(GcDCC_DCBMSBulkChrgTimeRest_min) -> GcDCC_DCBMSBulkChrgTimeRest_min/1

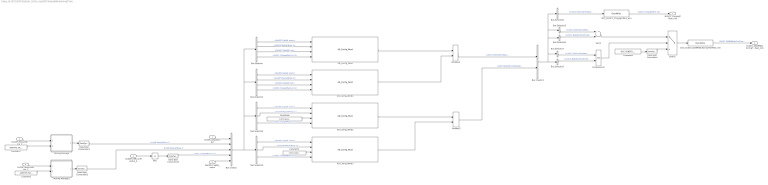
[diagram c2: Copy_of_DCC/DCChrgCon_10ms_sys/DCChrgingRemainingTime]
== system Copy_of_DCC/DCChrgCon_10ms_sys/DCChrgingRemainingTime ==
  GcSOC_DispSOC_pct : Inport
  GcCDP_MinCellTemp_C : Inport  Port=2
  GcGDP_CMLCurMaxOut_A : Inport  Port=3
  GcCDP_MaxCellTemp_C : Inport  Port=4
  GeUDS_CapSel_enum : Inport  Port=5
  4D_Config_Word{,1..3} (4 alike) : AIWAYS_Powertrain_BMS_lib/Signals/4D_Config_Word  Default_Cal_Breakpoint1_Name=CaDCC_CATL203TimeRestTempTable_C  Default_Cal_Breakpoint2_Name=CaDCC_CATL203TimeRestSOCTable_pct  Default_Cal_Breakpoint3_Name=CaDCC_CATL203TimeRestCMLCurrTable_A  Default_Cal_Table1_Name=CaDCC_CATL203DCChrgTimeRestTable_min  CATL153Ah_Cal_Breakpoint1_Name=CaDCC_CATL203TimeRestTempTable_C  CATL153Ah_Cal_Breakpoint2_Name=CaDCC_CATL203TimeRestSOCTable_pct  CATL153Ah_Cal_Breakpoint3_Name=CaDCC_CATL203TimeRestCMLCurrTable_A  CATL153Ah_Cal_Table1_Name=CaDCC_CATL203DCChrgTimeRestTable_min  CATL180Ah_Cal_Breakpoint1_Name=CaDCC_CATL203TimeRestTempTable_C  CATL180Ah_Cal_Breakpoint2_Name=CaDCC_CATL203TimeRestSOCTable_pct  CATL180Ah_Cal_Breakpoint3_Name=CaDCC_CATL203TimeRestCMLCurrTable_A  CATL180Ah_Cal_Table1_Name=CaDCC_CATL203DCChrgTimeRestTable_min  CATL177Ah_Cal_Breakpoint1_Name=CaDCC_CATL177TimeRestTempTable_C  CATL177Ah_Cal_Breakpoint2_Name=CaDCC_CATL177TimeRestSOCTable_pct  CATL177Ah_Cal_Breakpoint3_Name=CaDCC_CATL177TimeRestCMLCurrTable_A  CATL177Ah_Cal_Table1_Name=CaDCC_CATL177DCChrgTimeRestTable_min  CATL203Ah_Cal_Breakpoint1_Name=CaDCC_CATL203TimeRestTempTable_C  CATL203Ah_Cal_Breakpoint2_Name=CaDCC_CATL203TimeRestSOCTable_pct  CATL203Ah_Cal_Breakpoint3_Name=CaDCC_CATL203TimeRestCMLCurrTable_A  CATL203Ah_Cal_Table1_Name=CaDCC_CATL203DCChrgTimeRestTable_min  CATL51Ah_Cal_Breakpoint1_Name=CaDCC_CATL177TimeRestTempTable_C  CATL51Ah_Cal_Breakpoint2_Name=CaDCC_CATL177TimeRestSOCTable_pct  CATL51Ah_Cal_Breakpoint3_Name=CaDCC_CATL177TimeRestCMLCurrTable_A  CATL51Ah_Cal_Table1_Name=CaDCC_CATL177DCChrgTimeRestTable_min  CATL132Ah_Cal_Breakpoint1_Name=CaDCC_CATL177TimeRestTempTable_C  CATL132Ah_Cal_Breakpoint2_Name=CaDCC_CATL177TimeRestSOCTable_pct  CATL132Ah_Cal_Breakpoint3_Name=CaDCC_CATL177TimeRestCMLCurrTable_A  CATL132Ah_Cal_Table1_Name=CaDCC_CATL177DCChrgTimeRestTable_min  XWD75Ah_Cal_Breakpoint1_Name=CaDCC_XWD75TimeRestTempTable_C  XWD75Ah_Cal_Breakpoint2_Name=CaDCC_XWD75TimeRestSOCTable_pct  XWD75Ah_Cal_Breakpoint3_Name=CaDCC_XWD75TimeRestCMLCurrTable_A  XWD75Ah_Cal_Table1_Name=CaDCC_XWD75DCChrgTimeRestTable_min  TFE177Ah_Cal_Breakpoint1_Name=CaDCC_TFE177TimeRestTempTable_C  TFE177Ah_Cal_Breakpoint2_Name=CaDCC_TFE177TimeRestSOCTable_pct  TFE177Ah_Cal_Breakpoint3_Name=CaDCC_TFE177TimeRestCMLCurrTable_A  TFE177Ah_Cal_Table1_Name=CaDCC_TFE177DCChrgTimeRestTable_min  CATLCTP248Ah_Cal_Breakpoint1_Name=CaDCC_CATL177TimeRestTempTable_C  CATLCTP248Ah_Cal_Breakpoint2_Name=CaDCC_CATL177TimeRestSOCTable_pct  CATLCTP248Ah_Cal_Breakpoint3_Name=CaDCC_CATL177TimeRestCMLCurrTable_A  CATLCTP248Ah_Cal_Table1_Name=CaDCC_CATL177DCChrgTimeRestTable_min
  Abs : Abs
  Bus Creator : BusCreator  Inputs=5
  Bus Creator1 : BusCreator  Inputs=2
  Bus Selector : BusSelector  OutputSignals=GeUDS_CapSel_enum,GcCDP_MinCellTemp_C,GcSOC_DispSOC_pct,LcDCC_ChargerMaxCurr_A
  Bus Selector1 : BusSelector  OutputSignals=GeUDS_CapSel_enum,GcCDP_MaxCellTemp_C,GcSOC_DispSOC_pct,LcDCC_ChargerMaxCurr_A
  Bus Selector2 : BusSelector  OutputSignals=LcDCC_BulkSOCChrgTimeRest_min
  Bus Selector3 : BusSelector  OutputSignals=LcDCC_FullChrgTimeRest_min
  Bus Selector4 : BusSelector  OutputSignals=GeUDS_CapSel_enum,GcCDP_MaxCellTemp_C,LcDCC_ChargerMaxCurr_A
  Bus Selector5 : BusSelector  OutputSignals=GeUDS_CapSel_enum,GcCDP_MinCellTemp_C,LcDCC_ChargerMaxCurr_A
  Bus Selector6 : BusSelector  OutputSignals=LcDCC_FullChrgTimeRest_min
  Bus Selector7 : BusSelector  OutputSignals=LcDCC_FullChrgTimeRest_min
  Bus Selector8 : BusSelector  OutputSignals=LcDCC_BulkSOCChrgTimeRest_min
  Comparison1 : RelationalOperator  OutDataTypeStr=boolean
  Constant1 : Constant  Value=CcDCC_BulkSOC_pct
  Constant2 : Constant  Value=DCC_CONST0_NUMB
  Constant3 : Constant  Value=ASWTYPE_FALSE
  Constant6 : Constant  Value=CcDCC_BulkSOC_pct
  Constant7 : Constant  Value=ASWTYPE_FALSE
  DCC_GcDCC_ChrgingTiRem_min : AIWAYS_Powertrain_BMS_lib/Signals/OverWrite  OverWrite_Value=CcDCC_ChrgingTiRemOvr_min  OverWrite_flag=CbDCC_ChrgingTiRemOvrSwt_flg
  DCC_GcDCC_DCBMSBulkChrgTimeRest_min : AIWAYS_Powertrain_BMS_lib/Signals/OverWrite  OverWrite_Value=CcDCC_DCBMSBulkChrgTimeRestOvr_min  OverWrite_flag=CbDCC_DCBMSBulkChrgTimeRestOvrSwt_flg
  Data Type Conversion : DataTypeConversion
  Data Type Conversion1 : DataTypeConversion  OutDataTypeStr=fixdt(0,8,1,-40)  RndMeth=Round
  Data Type Conversion2 : DataTypeConversion  OutDataTypeStr=fixdt(0,8,1,-40)  RndMeth=Round
  Data Type Conversion3 : DataTypeConversion  OutDataTypeStr=uint16
  MinMax2 : MinMax  Function=max  Inputs=2  OutDataTypeStr=Inherit: Inherit via back propagation
  MinMax4 : MinMax  Function=max  Inputs=2  OutDataTypeStr=Inherit: Inherit via back propagation  RndMeth=Zero
  Moving Average : Subsystem  TreatAsAtomicUnit=on  mask(MovingAverage00){BufferSize=CcDCC_CellTempFilterAvg_numb}
      mask prompts: BufferSize "Buffer size"
      mask help: Block will compute the moving average of the input signal based on the number of samples input as the buffer_size. NOTE: Will not work with vectorized inputs. Default buffer size = 2. Input1=Value; Input2=Reset
  Moving Average1 : Subsystem  TreatAsAtomicUnit=on  mask(MovingAverage00){BufferSize=CcDCC_CellTempFilterAvg_numb}
      mask prompts: BufferSize "Buffer size"
      mask help: Block will compute the moving average of the input signal based on the number of samples input as the buffer_size. NOTE: Will not work with vectorized inputs. Default buffer size = 2. Input1=Value; Input2=Reset
  Sum1 : Sum  Inputs=+-  OutDataTypeStr=Inherit: Inherit via back propagation  RndMeth=Zero
  Switch : Switch  Criteria=u2 ~= 0  Threshold=1  RndMeth=Zero
  GcDCC_ChrgingTiRem_min : Outport
  GcDCC_DCBMSBulkChrgTimeRest_min : Outport  Port=2
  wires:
  DCC_GcDCC_ChrgingTiRem_min/1 -> GcDCC_ChrgingTiRem_min/1  "GcDCC_ChrgingTiRem_min"
  Bus Selector7/1 -> Comparison1/1  "<LcDCC_FullChrgTimeRest_min>"
  MinMax2/1 -> Bus Creator1/2  "LcDCC_BulkSOCChrgTimeRest_min"
  MinMax4/1 -> Bus Creator1/1  "LcDCC_FullChrgTimeRest_min"
  Bus Selector/4 -> 4D_Config_Word/4  "<LcDCC_ChargerMaxCurr_A>"
  Bus Creator/1 -> Bus Selector/1, Bus Selector1/1, Bus Selector4/1, Bus Selector5/1
  4D_Config_Word1/1 -> MinMax4/2
  4D_Config_Word2/1 -> MinMax2/1
  Bus Creator1/1 -> Bus Selector8/1, Bus Selector3/1, Bus Selector6/1, Bus Selector7/1, Bus Selector2/1
  Abs/1 -> Data Type Conversion3/1
  Bus Selector4/2 -> 4D_Config_Word2/2  "<GcCDP_MaxCellTemp_C>"
  Bus Selector4/3 -> 4D_Config_Word2/4  "<LcDCC_ChargerMaxCurr_A>"
  Bus Selector5/2 -> 4D_Config_Word3/2  "<GcCDP_MinCellTemp_C>"
  Constant6/1 -> 4D_Config_Word2/3
  Constant1/1 -> 4D_Config_Word3/3
  GcGDP_CMLCurMaxOut_A/1 -> Abs/1
  Bus Selector5/3 -> 4D_Config_Word3/4  "<LcDCC_ChargerMaxCurr_A>"
  Bus Selector/3 -> 4D_Config_Word/3  "<GcSOC_DispSOC_pct>"
  Bus Selector/2 -> 4D_Config_Word/2  "<GcCDP_MinCellTemp_C>"
  4D_Config_Word3/1 -> MinMax2/2
  GcSOC_DispSOC_pct/1 -> Bus Creator/1
  4D_Config_Word/1 -> MinMax4/1
  Bus Selector6/1 -> DCC_GcDCC_ChrgingTiRem_min/1  "<LcDCC_FullChrgTimeRest_min>"
  Bus Selector2/1 -> Comparison1/2  "<LcDCC_BulkSOCChrgTimeRest_min>"
  Comparison1/1 -> Switch/2
  Bus Selector3/1 -> Sum1/1  "<LcDCC_FullChrgTimeRest_min>"
  Bus Selector8/1 -> Sum1/2  "<LcDCC_BulkSOCChrgTimeRest_min>"
  Sum1/1 -> Switch/1
  Constant2/1 -> Data Type Conversion/1
  Data Type Conversion/1 -> Switch/3
  GeUDS_CapSel_enum/1 -> Bus Creator/5
  Bus Selector/1 -> 4D_Config_Word/1  "<GeUDS_CapSel_enum>"
  Bus Selector1/1 -> 4D_Config_Word1/1  "<GeUDS_CapSel_enum>"
  Bus Selector1/2 -> 4D_Config_Word1/2  "<GcCDP_MaxCellTemp_C>"
  Bus Selector1/3 -> 4D_Config_Word1/3  "<GcSOC_DispSOC_pct>"
  Bus Selector1/4 -> 4D_Config_Word1/4  "<LcDCC_ChargerMaxCurr_A>"
  Bus Selector4/1 -> 4D_Config_Word2/1  "<GeUDS_CapSel_enum>"
  Bus Selector5/1 -> 4D_Config_Word3/1  "<GeUDS_CapSel_enum>"
  Switch/1 -> DCC_GcDCC_DCBMSBulkChrgTimeRest_min/1
  DCC_GcDCC_DCBMSBulkChrgTimeRest_min/1 -> GcDCC_DCBMSBulkChrgTimeRest_min/1  "GcDCC_DCBMSBulkChrgTimeRest_min"
  Constant7/1 -> Moving Average/2(R)
  GcCDP_MinCellTemp_C/1 -> Moving Average/1(u)
  Moving Average/1(y) -> Data Type Conversion1/1
  Constant3/1 -> Moving Average1/2(R)
  GcCDP_MaxCellTemp_C/1 -> Moving Average1/1(u)
  Moving Average1/1(y) -> Data Type Conversion2/1
  Data Type Conversion1/1 -> Bus Creator/2  "GcCDP_MinCellTemp_C"
  Data Type Conversion2/1 -> Bus Creator/3  "GcCDP_MaxCellTemp_C"
  Data Type Conversion3/1 -> Bus Creator/4  "LcDCC_ChargerMaxCurr_A"

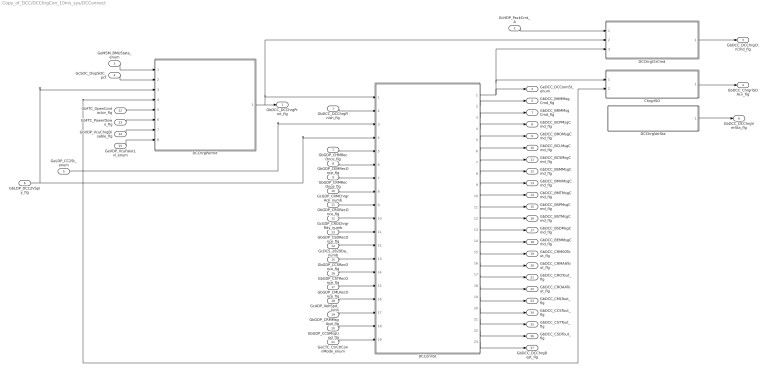
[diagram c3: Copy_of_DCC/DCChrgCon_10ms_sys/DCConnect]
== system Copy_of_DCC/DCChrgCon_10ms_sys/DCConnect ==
  GbDCC_DCChrgFinish_flg : Inport
  GcHDP_PackCrnt_A : Inport  Port=2
  GeMSM_BMUState_enum : Inport  Port=3
  GcSOC_DispSOC_pct : Inport  Port=4
  GeLDP_CC2St_enum : Inport  Port=5
  GbLDP_DC12VSply_flg : Inport  Port=6
  GbGDP_CHMRecOnce_flg : Inport  Port=7
  GbGDP_CEMRecOnce_flg : Inport  Port=8
  GbGDP_CRMRecOnce_flg : Inport  Port=9
  GcGDP_CRMChrgrAck_numb : Inport  Port=10
  GbGDP_CRORecOnce_flg : Inport  Port=11
  GcGDP_CROChrgrRdy_numb : Inport  Port=12
  GbGDP_CSDRecOnce_flg : Inport  Port=13
  GcDCS_2829Da_numb : Inport  Port=14
  GbGDP_CCSRecOnce_flg : Inport  Port=15
  GbGDP_CSTRecOnce_flg : Inport  Port=16
  GbGDP_CMLRecOnce_flg : Inport  Port=17
  GcADP_VehSpd_kmh : Inport  Port=18
  GbGDP_CRMMsgUpd_flg : Inport  Port=19
  GbGDP_CCSMsgUpd_flg : Inport  Port=20
  GeCTC_CtrCtlConnMode_enum : Inport  Port=21
  GbFTC_OpenContactor_flg : Inport  Port=22
  GbFTC_PowerDown_flg : Inport  Port=23
  GbVDP_VcuChrgDisable_flg : Inport  Port=24
  GeVDP_VcuFalutLvl_enum : Inport  Port=25
  ChrgrISO : Subsystem
  DCChrgCtrCmd : Subsystem
  DCChrgPermit : Subsystem
  DCChrgVerSta : Subsystem
  DCConnSt : Subsystem
  GbDCC_DCChrgPrmt_flg : Outport
  GeDCC_DCConnSt_enum : Outport  Port=2
  GbDCC_DCChrgCtrCmd_flg : Outport  Port=3
  GbDCC_ChrgrISOAcv_flg : Outport  Port=4
  GbDCC_BHMMsgCmd_flg : Outport  Port=5
  GbDCC_DCChrgVerSta_flg : Outport  Port=6
  GbDCC_BRMMsgCmd_flg : Outport  Port=7
  GbDCC_BCPMsgCmd_flg : Outport  Port=8
  GbDCC_BROMsgCmd_flg : Outport  Port=9
  GbDCC_BCLMsgCmd_flg : Outport  Port=10
  GbDCC_BCSMsgCmd_flg : Outport  Port=11
  GbDCC_BSMMsgCmd_flg : Outport  Port=12
  GbDCC_BMVMsgCmd_flg : Outport  Port=13
  GbDCC_BMTMsgCmd_flg : Outport  Port=14
  GbDCC_BSPMsgCmd_flg : Outport  Port=15
  GbDCC_BSTMsgCmd_flg : Outport  Port=16
  GbDCC_BSDMsgCmd_flg : Outport  Port=17
  GbDCC_BEMMsgCmd_flg : Outport  Port=18
  GbDCC_CRM00Tout_flg : Outport  Port=19
  GbDCC_CRMAATout_flg : Outport  Port=20
  GbDCC_CROTout_flg : Outport  Port=21
  GbDCC_CROAATout_flg : Outport  Port=22
  GbDCC_CMLTout_flg : Outport  Port=23
  GbDCC_CCSTout_flg : Outport  Port=24
  GbDCC_CSTTout_flg : Outport  Port=25
  GbDCC_CSDTout_flg : Outport  Port=26
  GbDCC_DCChrgRqst_flg : Outport  Port=27
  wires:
  GcHDP_PackCrnt_A/1 -> DCChrgCtrCmd/1(GcHDP_PackCrnt_A)
  DCChrgPermit/1(GbDCC_DCChrgPrmt_flg) -> DCChrgCtrCmd/2(GbDCC_DCChrgPrmt_flg), DCConnSt/1(GbDCC_DCChrgPrmt_flg), GbDCC_DCChrgPrmt_flg/1
  DCConnSt/6(GbDCC_BCLMsgCmd_flg) -> GbDCC_BCLMsgCmd_flg/1
  DCConnSt/5(GbDCC_BROMsgCmd_flg) -> GbDCC_BROMsgCmd_flg/1
  DCConnSt/13(GbDCC_BSDMsgCmd_flg) -> GbDCC_BSDMsgCmd_flg/1
  DCConnSt/22(GbDCC_CSDTout_flg) -> GbDCC_CSDTout_flg/1
  DCConnSt/14(GbDCC_BEMMsgCmd_flg) -> GbDCC_BEMMsgCmd_flg/1
  DCConnSt/9(GbDCC_BMVMsgCmd_flg) -> GbDCC_BMVMsgCmd_flg/1
  DCConnSt/15(GbDCC_CRM00Tout_flg) -> GbDCC_CRM00Tout_flg/1
  DCConnSt/20(GbDCC_CCSTout_flg) -> GbDCC_CCSTout_flg/1
  DCConnSt/4(GbDCC_BCPMsgCmd_flg) -> GbDCC_BCPMsgCmd_flg/1
  DCConnSt/11(GbDCC_BSPMsgCmd_flg) -> GbDCC_BSPMsgCmd_flg/1
  DCConnSt/2(GbDCC_BHMMsgCmd_flg) -> GbDCC_BHMMsgCmd_flg/1
  DCConnSt/17(GbDCC_CROTout_flg) -> GbDCC_CROTout_flg/1
  DCConnSt/21(GbDCC_CSTTout_flg) -> GbDCC_CSTTout_flg/1
  DCConnSt/19(GbDCC_CMLTout_flg) -> GbDCC_CMLTout_flg/1
  DCConnSt/18(GbDCC_CROAATout_flg) -> GbDCC_CROAATout_flg/1
  DCConnSt/8(GbDCC_BSMMsgCmd_flg) -> GbDCC_BSMMsgCmd_flg/1
  DCConnSt/3(GbDCC_BRMMsgCmd_flg) -> GbDCC_BRMMsgCmd_flg/1
  DCConnSt/7(GbDCC_BCSMsgCmd_flg) -> GbDCC_BCSMsgCmd_flg/1
  DCConnSt/1(GeDCC_DCConnSt_enum) -> ChrgrISO/1(GeDCC_DCConnSt_enum), DCChrgCtrCmd/3(GeDCC_DCConnSt_enum), GeDCC_DCConnSt_enum/1
  DCConnSt/12(GbDCC_BSTMsgCmd_flg) -> GbDCC_BSTMsgCmd_flg/1
  DCConnSt/16(GbDCC_CRMAATout_flg) -> GbDCC_CRMAATout_flg/1
  DCConnSt/10(GbDCC_BMTMsgCmd_flg) -> GbDCC_BMTMsgCmd_flg/1
  DCChrgVerSta/1(GbDCC_DCChrgVerSta_flg) -> GbDCC_DCChrgVerSta_flg/1
  DCChrgCtrCmd/1(GbDCC_DCChrgCtrCmd_flg) -> GbDCC_DCChrgCtrCmd_flg/1
  GeMSM_BMUState_enum/1 -> DCChrgPermit/1(GeMSM_BMUState_enum)
  GbLDP_DC12VSply_flg/1 -> DCChrgPermit/3(GbLDP_DC12VSply_flg), DCConnSt/4(GbLDP_DC12VSply_flg)
  ChrgrISO/1(GbDCC_ChrgrISOAcv_flg) -> GbDCC_ChrgrISOAcv_flg/1
  GcSOC_DispSOC_pct/1 -> DCChrgPermit/2(GcSOC_DispSOC_pct)
  GeLDP_CC2St_enum/1 -> ChrgrISO/2(GeLDP_CC2St_enum), DCConnSt/3(GeLDP_CC2St_enum), DCChrgPermit/4(GeLDP_CC2St_enum)
  GbDCC_DCChrgFinish_flg/1 -> DCConnSt/2(GbDCC_DCChrgFinish_flg)
  GbGDP_CHMRecOnce_flg/1 -> DCConnSt/5(GbGDP_CHMRecOnce_flg)
  GbGDP_CEMRecOnce_flg/1 -> DCConnSt/6(GbGDP_CEMRecOnce_flg)
  GbGDP_CRMRecOnce_flg/1 -> DCConnSt/7(GbGDP_CRMRecOnce_flg)
  GcGDP_CRMChrgrAck_numb/1 -> DCConnSt/8(GcGDP_CRMChrgrAck_numb)
  GbGDP_CRORecOnce_flg/1 -> DCConnSt/9(GbGDP_CRORecOnce_flg)
  GcGDP_CROChrgrRdy_numb/1 -> DCConnSt/10(GcGDP_CROChrgrRdy_numb)
  GbGDP_CSDRecOnce_flg/1 -> DCConnSt/11(GbGDP_CSDRecOnce_flg)
  GcDCS_2829Da_numb/1 -> DCConnSt/12(GcDCS_2829Da_numb)
  GbGDP_CCSRecOnce_flg/1 -> DCConnSt/13(GbGDP_CCSRecOnce_flg)
  GbGDP_CSTRecOnce_flg/1 -> DCConnSt/14(GbGDP_CSTRecOnce_flg)
  GbGDP_CMLRecOnce_flg/1 -> DCConnSt/15(GbGDP_CMLRecOnce_flg)
  GcADP_VehSpd_kmh/1 -> DCConnSt/16(GcADP_VehSpd_kmh)
  GbGDP_CRMMsgUpd_flg/1 -> DCConnSt/17(GbGDP_CRMMsgUpd_flg)
  GbGDP_CCSMsgUpd_flg/1 -> DCConnSt/18(GbGDP_CCSMsgUpd_flg)
  GeCTC_CtrCtlConnMode_enum/1 -> DCConnSt/19(GeCTC_CtrCtlConnMode_enum)
  GbFTC_OpenContactor_flg/1 -> DCChrgPermit/5(GbFTC_OpenContactor_flg)
  GbFTC_PowerDown_flg/1 -> DCChrgPermit/6(GbFTC_PowerDown_flg)
  GbVDP_VcuChrgDisable_flg/1 -> DCChrgPermit/7(GbVDP_VcuChrgDisable_flg)
  GeVDP_VcuFalutLvl_enum/1 -> DCChrgPermit/8(GeVDP_VcuFalutLvl_enum)
  DCConnSt/23(GbDCC_DCChrgRqst_flg) -> GbDCC_DCChrgRqst_flg/1

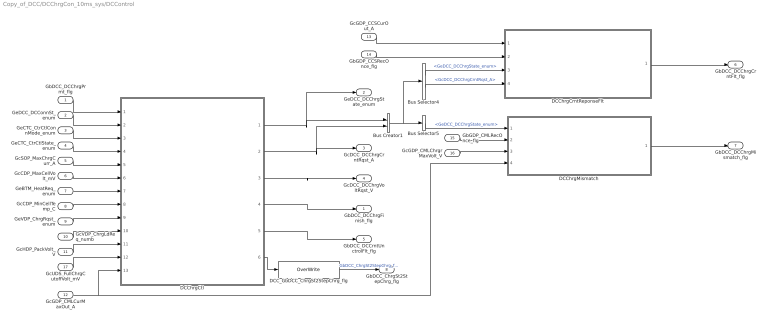
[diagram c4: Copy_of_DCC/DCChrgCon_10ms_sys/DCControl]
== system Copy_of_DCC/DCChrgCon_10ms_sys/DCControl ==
  GbDCC_DCChrgPrmt_flg : Inport
  GeDCC_DCConnSt_enum : Inport  Port=2
  GeCTC_CtrCtlConnMode_enum : Inport  Port=3
  GeCTC_CtrCtlState_enum : Inport  Port=4
  GcSOP_MaxChrgCurr_A : Inport  Port=5
  GcCDP_MaxCellVolt_mV : Inport  Port=6
  GeBTM_HeatReq_enum : Inport  Port=7
  GcCDP_MinCellTemp_C : Inport  Port=8
  GeVDP_ChrgRqst_enum : Inport  Port=9
  GcVDP_ChrgLdReq_numb : Inport  Port=10
  GcHDP_PackVolt_V : Inport  Port=11
  GcGDP_CMLCurMaxOut_A : Inport  Port=12
  GcGDP_CCSCurOut_A : Inport  Port=13
  GbGDP_CCSRecOnce_flg : Inport  Port=14
  GbGDP_CMLRecOnce_flg : Inport  Port=15
  GcGDP_CMLChrgrMaxVolt_V : Inport  Port=16
  GcUDS_FullChrgCutoffVolt_mV : Inport  Port=17
  Bus Creator1 : BusCreator  Inputs=2
  Bus Selector4 : BusSelector  OutputSignals=GeDCC_DCChrgState_enum,GcDCC_DCChrgCrntRqst_A
  Bus Selector5 : BusSelector  OutputSignals=GeDCC_DCChrgState_enum
  DCC_GbDCC_ChrgSt2StepChrg_flg : AIWAYS_Powertrain_BMS_lib/Signals/OverWrite  OverWrite_Value=CbDCC_ChrgSt2StepChrgOvr_flg  OverWrite_flag=CbDCC_ChrgSt2StepChrgOvrSwt_flg
  DCChrgCrntReponseFlt : Subsystem
  DCChrgCtl : Subsystem
  DCChrgMismatch : Subsystem
  GbDCC_DCChrgFinish_flg : Outport
  GeDCC_DCChrgState_enum : Outport  Port=2
  GcDCC_DCChrgCrntRqst_A : Outport  Port=3
  GcDCC_DCChrgVoltRqst_V : Outport  Port=4
  GbDCC_DCCrntUnctrolFlt_flg : Outport  Port=5
  GbDCC_DCChrgCrntFlt_flg : Outport  Port=6
  GbDCC_DCChrgMismatch_flg : Outport  Port=7
  GbDCC_ChrgSt2StepChrg_flg : Outport  Port=8
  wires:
  GcGDP_CMLChrgrMaxVolt_V/1 -> DCChrgMismatch/3(GcGDP_CMLChrgrMaxVolt_V)
  GbGDP_CMLRecOnce_flg/1 -> DCChrgMismatch/2(GbGDP_CMLRecOnce_flg)
  GcGDP_CMLCurMaxOut_A/1 -> DCChrgMismatch/4(GcGDP_CMLCurMaxOut_A), DCChrgCtl/13(GcGDP_CMLCurMaxOut_A)
  DCChrgCtl/2(GcDCC_DCChrgCrntRqst_A) -> GcDCC_DCChrgCrntRqst_A/1, Bus Creator1/2
  DCChrgCrntReponseFlt/1(GbDCC_DCChrgCrntFlt_flg) -> GbDCC_DCChrgCrntFlt_flg/1
  DCChrgCtl/1(GeDCC_DCChrgState_enum) -> Bus Creator1/1, GeDCC_DCChrgState_enum/1
  Bus Selector4/2 -> DCChrgCrntReponseFlt/4(GcDCC_DCChrgCrntRqst_A)  "<GcDCC_DCChrgCrntRqst_A>"
  Bus Selector4/1 -> DCChrgCrntReponseFlt/3(GeDCC_DCChrgState_enum)  "<GeDCC_DCChrgState_enum>"
  Bus Selector5/1 -> DCChrgMismatch/1(GeDCC_DCChrgState_enum)  "<GeDCC_DCChrgState_enum>"
  DCChrgMismatch/1(GbDCC_DCChrgMismatch_flg) -> GbDCC_DCChrgMismatch_flg/1
  Bus Creator1/1 -> Bus Selector4/1, Bus Selector5/1
  DCChrgCtl/5(GbDCC_DCCrntUnctrolFlt_flg) -> GbDCC_DCCrntUnctrolFlt_flg/1
  DCChrgCtl/3(GcDCC_DCChrgVoltRqst_V) -> GcDCC_DCChrgVoltRqst_V/1
  DCChrgCtl/4(GbDCC_DCChrgFinish_flg) -> GbDCC_DCChrgFinish_flg/1
  GbDCC_DCChrgPrmt_flg/1 -> DCChrgCtl/1(GbDCC_DCChrgPrmt_flg)
  GeDCC_DCConnSt_enum/1 -> DCChrgCtl/2(GeDCC_DCConnSt_enum)
  GeCTC_CtrCtlConnMode_enum/1 -> DCChrgCtl/3(GeCTC_CtrCtlConnMode_enum)
  GeCTC_CtrCtlState_enum/1 -> DCChrgCtl/4(GeCTC_CtrCtlState_enum)
  GcSOP_MaxChrgCurr_A/1 -> DCChrgCtl/5(GcSOP_MaxChrgCurr_A)
  GcCDP_MaxCellVolt_mV/1 -> DCChrgCtl/6(GcCDP_MaxCellVolt_mV)
  GeBTM_HeatReq_enum/1 -> DCChrgCtl/7(GeBTM_HeatReq_enum)
  GcCDP_MinCellTemp_C/1 -> DCChrgCtl/8(GcCDP_MinCellTemp_C)
  GeVDP_ChrgRqst_enum/1 -> DCChrgCtl/9(GeVDP_ChrgRqst_enum)
  GcVDP_ChrgLdReq_numb/1 -> DCChrgCtl/10(GcVDP_ChrgLdReq_numb)
  GcHDP_PackVolt_V/1 -> DCChrgCtl/11(GcHDP_PackVolt_V)
  GcGDP_CCSCurOut_A/1 -> DCChrgCrntReponseFlt/1(GcGDP_CCSCurOut_A)
  GbGDP_CCSRecOnce_flg/1 -> DCChrgCrntReponseFlt/2(GbGDP_CCSRecOnce_flg)
  DCChrgCtl/6(LbDCC_ChrgSt2StepChrg_flg) -> DCC_GbDCC_ChrgSt2StepChrg_flg/1
  DCC_GbDCC_ChrgSt2StepChrg_flg/1 -> GbDCC_ChrgSt2StepChrg_flg/1  "GbDCC_ChrgSt2StepChrg_flg"
  GcUDS_FullChrgCutoffVolt_mV/1 -> DCChrgCtl/12(GcUDS_FullChrgCutoffVolt_mV)

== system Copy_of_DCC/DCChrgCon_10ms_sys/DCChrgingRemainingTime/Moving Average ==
  note: Moving Average
  u : Inport
  R : Inport  Port=2  OutDataTypeStr=boolean
  Chart : Stateflow chart  TreatAsAtomicUnit=on
  Signal Conversion : SignalConversion  ConversionOutput=Contiguous copy  OverrideOpt=off
  y : Outport
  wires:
  Signal Conversion/1 -> y/1
  Chart/1(Y) -> Signal Conversion/1
  u/1 -> Chart/1(u)
  R/1 -> Chart/2(R)

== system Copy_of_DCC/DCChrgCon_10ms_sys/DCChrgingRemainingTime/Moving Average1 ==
  note: Moving Average
  u : Inport
  R : Inport  Port=2  OutDataTypeStr=boolean
  Chart : Stateflow chart  TreatAsAtomicUnit=on
  Signal Conversion : SignalConversion  ConversionOutput=Contiguous copy  OverrideOpt=off
  y : Outport
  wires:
  R/1 -> Chart/2(R)
  u/1 -> Chart/1(u)
  Chart/1(Y) -> Signal Conversion/1
  Signal Conversion/1 -> y/1

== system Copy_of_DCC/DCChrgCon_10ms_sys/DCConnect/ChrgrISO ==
  GeDCC_DCConnSt_enum : Inport
  GeLDP_CC2St_enum : Inport  Port=2
  BMSDelay : AIWAYS_Powertrain_BMS_lib/Debounce & Delay/BMSDelay
  Constant : Constant  Value=ASWTYPE_FALSE
  Constant1 : Constant  Value=Enum_DCCDCConnSt.Enum_DCCDCConnSt_HandShake
  Constant2 : Constant  Value=Enum_DCCDCConnSt.Enum_DCCDCConnSt_ID
  Constant3 : Constant  Value=Enum_DCCDCConnSt.Enum_DCCDCConnSt_CFG
  Constant4 : Constant  Value=Enum_LDPCC2St.Enum_LDPCC2St_Connect
  Constant5 : Constant  Value=Enum_DCCDCConnSt.Enum_DCCDCConnSt_Default
  Constant6 : Constant  Value=DCC_RUNTIME_MS
  Constant7 : Constant  Value=CcDCC_IsoDisableDelay_ms
  DCC1_GbDCC_ChrgrISOAcv_flg : AIWAYS_Powertrain_BMS_lib/Signals/OverWrite  OverWrite_Value=CbDCC_ChrgrISOAcvOvr_flg  OverWrite_flag=CbDCC_ChrgrISOAcvOvrSwt_flg
  Data Type Conversion2 : DataTypeConversion
  Data Type Conversion4 : DataTypeConversion
  Logical Operator : Logic  Operator=OR  Inputs=4  AllPortsSameDT=off  OutDataTypeStr=boolean
  Logical Operator1 : Logic  AllPortsSameDT=off  OutDataTypeStr=boolean
  Logical Operator2 : Logic  AllPortsSameDT=off  OutDataTypeStr=boolean
  Relational Operator{1..6} (6 alike) : RelationalOperator  Operator===  OutDataTypeStr=boolean
  GbDCC_ChrgrISOAcv_flg : Outport
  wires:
  Logical Operator/1 -> DCC1_GbDCC_ChrgrISOAcv_flg/1
  Constant1/1 -> Relational Operator1/2
  GeDCC_DCConnSt_enum/1 -> Data Type Conversion4/1
  Constant2/1 -> Relational Operator2/2
  Constant3/1 -> Relational Operator3/2
  Relational Operator1/1 -> Logical Operator/1
  Relational Operator2/1 -> Logical Operator/2
  Relational Operator3/1 -> Logical Operator/3
  DCC1_GbDCC_ChrgrISOAcv_flg/1 -> GbDCC_ChrgrISOAcv_flg/1  "GbDCC_ChrgrISOAcv_flg"
  Data Type Conversion4/1 -> Relational Operator1/1, Relational Operator2/1, Relational Operator3/1, Relational Operator5/1
  Data Type Conversion2/1 -> Relational Operator4/1
  Relational Operator4/1 -> Logical Operator1/2
  Constant4/1 -> Relational Operator4/2
  GeLDP_CC2St_enum/1 -> Data Type Conversion2/1
  Constant5/1 -> Relational Operator5/2
  Relational Operator5/1 -> Logical Operator1/1
  Logical Operator1/1 -> Logical Operator2/2, BMSDelay/1
  Constant6/1 -> BMSDelay/2
  Constant7/1 -> BMSDelay/3
  Logical Operator2/1 -> Logical Operator/4
  BMSDelay/1 -> Relational Operator6/1
  Relational Operator6/1 -> Logical Operator2/1
  Constant/1 -> Relational Operator6/2
